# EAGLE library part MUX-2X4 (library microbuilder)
2x4 Channel Analog Multiplexer/Demultiplexer [Part No.] Texas Instruments CD74HC4052M Digikey: 296-9218-5-ND
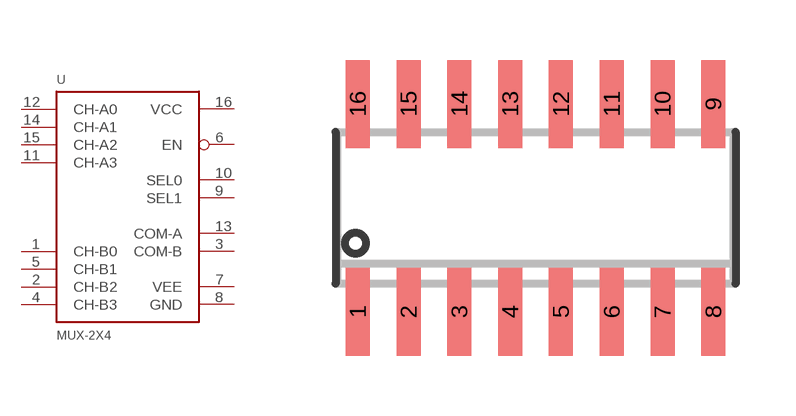
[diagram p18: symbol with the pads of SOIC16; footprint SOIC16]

Designator prefix U

## MUX-2X4  [SOIC16]
1  CH-B0
2  CH-B2
3  COM-B
4  CH-B3
5  CH-B1
6  EN
7  VEE
8  GND
9  SEL1
10  SEL0
11  CH-A3
12  CH-A0
13  COM-A
14  CH-A1
15  CH-A2
16  VCC

## Footprint SOIC16 (pad centres in mm)
SMALL OUTLINE INTEGRATED CIRCUIT
smd 0.6 x 2.2: 1 -4.445,-2.6; 2 -3.175,-2.6; 3 -1.905,-2.6; 4 -0.635,-2.6; 5 0.635,-2.6; 6 1.905,-2.6; 7 3.175,-2.6; 8 4.445,-2.6; 9 4.445,2.6; 10 3.175,2.6; 11 1.905,2.6; 12 0.635,2.6; 13 -0.635,2.6; 14 -1.905,2.6; 15 -3.175,2.6; 16 -4.445,2.6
